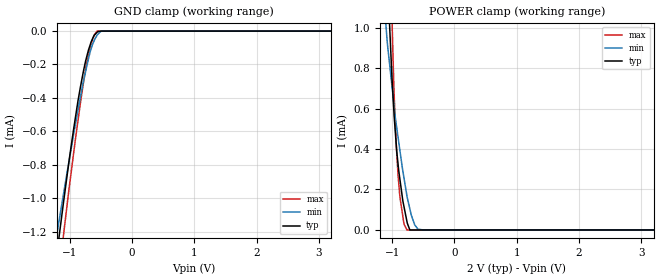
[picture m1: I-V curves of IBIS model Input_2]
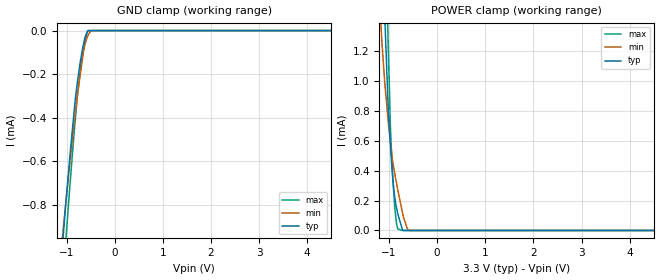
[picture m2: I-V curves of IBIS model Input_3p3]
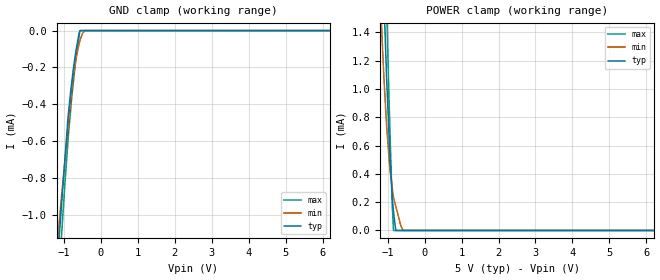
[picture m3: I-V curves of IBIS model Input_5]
|Texas Instruments Incorporated
|12-Bit, Octal, Ultralow Glitch, Voltage Output Digital to Analog Converter
| Marketing part#   Digital Voltage Range   Package-type   #pins
| DAC7558IRHBR   2.7 to 5.5V   QFN   32
| DAC7558IRHBRG4   2.7 to 5.5V   QFN   32
| DAC7558IRHBT   2.7 to 5.5V   QFN   32
| DAC7558IRHBTG4   2.7 to 5.5V   QFN   32
[IBIS Ver]   3.2
[File name]   dac7558.ibs
|SIMDE Ver   V2.0 - 201002 - RHL4 - Build 372
[File Rev]   1.1
[Date]   August 03, 2010
[Source]
|   Texas Instruments Incorporated.
|   Analog-eLab Design Center, HPA
|   12500 TI Blvd
|   Dallas, TX -75243
|   e-mail: elab_ibis@list.ti.com
|   -Model generated from simulations in TISPICE
[Notes]   Revision History:
|   Rev 1.0: 07/13/2010
|   - Initial version of the model
|   - Model generated from simulations in TISPICE
|   - Model matched to SPICE simulation
|   - Models with names containing a trailing 3p3 contain
|   the models for 3.3V [3.0V and 3.6V]. Models with names
|   with trailing 5 contain the models for 5.0V [4.5V and
|   5.5V] operation. And Models with names containing trailing
|   2 contain models for 2V [1.8V and 2.2V].
|   - C_comp although listed in numerical order of value are
|   obtained from varying PVT conditions. For PVT conditions for
|   each specific value refer the buffer description under
|   respective [Model]. IBIS model user is responsible for using
|   appropriate C_comp to simulate for Signal Integrity.
|   Rev 1.1: 08/03/2010
|   - Corrected details under [Package] section.
|   - Added [Model Spec] in all input models
|   - Added comments for C_comp and [Temperature Range].
|   - Added C_comp for ON and HIGH IMPEDANCE states for
|   all 3-state buffers.
|   - Corrected Vinl and Vinh values in Input_3p3 and Input_5
|   models as per datasheet.
|   - Removed extra data points beyond -VDDtyp & 2*VDDtyp in
|   IV data.
|   - Corrected I-V/V-t mismatches for output models.
|   - Voltage range and Power clamp range for TERM changed to
|   1.8v to 5.5v
[Disclaimer]
| This model is designed as an aid for customers of Texas Instruments.
| TI and its licensors and suppliers make no warranties, either expressed
| or implied, with respect to this  model, including the warranties of
| merchantability or fitness for a particular purpose. The model is
| provided solely on an "as is" basis. The entire risk as to its quality
| and performance is with the customer.
[Copyright]
|(C) Copyright 2010 Texas Instruments Incorporated.All rights reserved.
|   DAC7558
[Component]   DAC7558
[Manufacturer]  TI
[Package]   | 32 QFN - RHB Package
|   typ   min   max
R_pkg   0.06441   0.03921   0.07733
L_pkg   1.08058nH   0.96917nH   1.25858nH
C_pkg   0.11700pF   0.10514pF   0.14494pF
|-------------------------PINS------------------------------------------------
[Pin]  signal_name model_name   R_pin   L_pin   C_pin
1   VFBA   TERM   0.07176   1.15274nH   0.10934pF
2   VOUTA   NC   0.06437   1.01850nH   0.10917pF
3   VOUTB   NC   0.06397   1.01087nH   0.10804pF
4   VFBB   TERM   0.06152   0.96917nH   0.10514pF
5   VFBC   TERM   0.06152   0.96920nH   0.10518pF
6   VOUTC   NC   0.06450   1.02377nH   0.10878pF
7   VOUTD   NC   0.06495   1.03230nH   0.11002pF
8   VFBD   TERM   0.07270   1.17584nH   0.11059pF
9   VREF2   NC   0.03936   0.98832nH   0.14273pF
10   SDO   OUTPUT   0.07733   1.25858nH   0.12438pF
11   IOVDD   POWER   0.03721   0.90944nH   0.14943pF
12   DGND   GND   0.03782   0.92935nH   0.14861pF
13   SDIN   INPUT   0.07429   1.20279nH   0.11973pF
14   SCLK   INPUT   0.07311   1.18150nH   0.11929pF
15   _SYNC   INPUT   0.07480   1.21269nH   0.12223pF
16   VREF3   NC   0.03924   0.98339nH   0.14461pF
17   VFBE   TERM   0.07270   1.17584nH   0.11064pF
18   VOUTE   NC   0.06495   1.03229nH   0.11003pF
19   VOUTF   NC   0.06450   1.02377nH   0.10879pF
20   VFBF   TERM   0.06152   0.96920nH   0.10518pF
21   VFBG   TERM   0.06152   0.96917nH   0.10514pF
22   VOUTG   NC   0.06397   1.01088nH   0.10803pF
23   VOUTH   NC   0.06437   1.01851nH   0.10917pF
24   VFBH   TERM   0.07176   1.15274nH   0.10941pF
25   VREF4   NC   0.03921   0.97897nH   0.14445pF
26   DCEN   INPUT   0.07480   1.20388nH   0.12194pF
27   _PD   INPUT   0.07311   1.17249nH   0.11840pF
28   VDD   POWER   0.03582   0.84776nH   0.15059pF
29   AGND   GND   0.02469   0.77509nH   0.17946pF
30   RSTSEL   INPUT   0.07315   1.17310nH   0.11837pF
31   _RST   INPUT   0.07509   1.20907nH   0.12231pF
32   VREF1   NC   0.03945   0.98680nH   0.14494pF
|   Model Selectors
[Model Selector]   INPUT
Input_2   2.0V digital input
Input_3p3   3.3V digital input
Input_5   5.0V digital input
[Model Selector]   OUTPUT
Output_2   2.0V digital tristate output
Output_3p3   3.3V digital tristate output
Output_5   5.0V digital tristate output
|   TERM Model
[Model] TERM
Model_type Terminator
C_comp   1.0e-20F   1.0e-20F   1.0e-20F
| variable   typ   min   max
[Voltage Range]   3.3V   1.8V   5.5V
[POWER Clamp Reference]  3.3V   1.8V   5.5V
[GND Clamp Reference]   0.0V   0.0V   0.0V
|Operating Temperature
|Ambient Temperature   25   105   -40
|Junction Temperature
[Temperature Range]   25   105   -40
| Models and submodels in the file (7): Input_2 (Input), Input_3p3 (Input), Input_5 (Input), Output_2 (3-state), Output_3p3 (3-state), Output_5 (3-state), TERM (Terminator)
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|   INPUT 2.0V Model
[Model]   Input_2
Model_type   Input
Vinl = 0
Vinh = 2.0
|   typ   min   max
|   (nom PVT)   (fast PVT)  (slow PVT)
|Average
C_comp   5.289e-13   5.087e-13   5.331e-13
|Where nom PVT is Nominal Process, 2V, 25C
|   fast PVT is Strong Process, 2.2V, -40C
|   slow PVT is Weak Process, 1.8V, 105C
[Model Spec]
Vinl   0   0   0
Vinh   2.0   1.8   2.2
[Voltage Range]   2   1.8   2.2
|Ambient Temperature   25   105   -40
|Junction Temperature
[Temperature Range]   25   105   -40
[Power Clamp Reference]   2   1.8   2.2
[GND Clamp Reference]   0   0   0
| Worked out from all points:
|   GND clamp passes 1 mA (typ) near -1.09 V on its own axis
|   POWER clamp passes 1 mA (typ) near -1.04 V on its own axis
[GND Clamp]
|   Voltage   I(typ)   I(min)   I(max)
-2V       -3.773mA   -3.073mA   -4.859mA
-1.198V   -1.313mA   -1.199mA   -1.559mA
-1.166V   -1.22mA    -1.127mA   -1.446mA
-1.096V   -1.017mA   -969.5uA   -1.211mA
-996mV    -740.9uA   -748.6uA   -904.1uA
-868mV    -421.9uA   -476.5uA   -540.8uA
-759.2mV  -205.8uA   -268.6uA   -262.6uA
-719.6mV  -144.4uA   -201.6uA   -175.3uA
-660.2mV  -71.04uA   -111.3uA   -82.3uA
-558.2mV  -6.611uA   -23.75uA   0A
-462.8mV  0A         0A         0A
4V        0A         0A         0A
[POWER Clamp]
|   Voltage   I(typ)   I(min)   I(max)
-2V       12.81mA    9.404mA    16.72mA
-1.098V   1.46mA     1.003mA    2.207mA
-1.052V   1.086mA    850.6uA    1.616mA
-1.025V   904.8uA    774.5uA    1.291mA
-1.002V   747.7uA    707.6uA    1.032mA
-957.2mV  517.2uA    579.4uA    580.3uA
-904.4mV  322.3uA    456.1uA    266.6uA
-809.8mV  114.9uA    256.2uA    29.07uA
-761.6mV  40.2uA     166.2uA    0A
-637.4mV  0A         24.9uA     0A
-491.6mV  0A         0A         0A
4V        0A         0A         0A
|   INPUT 3.3V Model
[Model]   Input_3p3
Model_type   Input
Vinl = 0.99
Vinh = 2.31
|   typ   min   max
|   (nom PVT)   (fast PVT)  (slow PVT)
|Average
C_comp   5.026e-13   4.615e-13   5.117e-13
|Where nom PVT is Nominal Process, 3.3V, 25C
|   fast PVT is Strong Process, 3.6V, -40C
|   slow PVT is Weak Process, 3.0V, 105C
[Model Spec]
Vinl   0.99   0.9   1.08
Vinh   2.31   2.1   2.52
[Voltage Range]   3.3   3   3.6
|Ambient Temperature   25   105   -40
|Junction Temperature
[Temperature Range]   25   105   -40
[Power Clamp Reference]   3.3   3   3.6
[GND Clamp Reference]   0   0   0
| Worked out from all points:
|   GND clamp passes 1 mA (typ) near -1.09 V on its own axis
|   POWER clamp passes 1 mA (typ) near -1.04 V on its own axis
[GND Clamp]
|   Voltage   I(typ)   I(min)   I(max)
-3.3V     -7.87mA    -6.18mA    -10.49mA
-1.136V   -1.137mA   -1.06mA    -1.344mA
-1.043V   -869.1uA   -851.3uA   -1.043mA
-1.016V   -796uA     -793uA     -965.3uA
-927.6mV  -570.2uA   -602.2uA   -704.9uA
-825mV    -329.3uA   -390.9uA   -425.6uA
-772.2mV  -232.4uA   -297.8uA   -290.7uA
-697.2mV  -121.4uA   -173.8uA   -154.5uA
-645mV    -59.97uA   -92.43uA   -82.6uA
-554.4mV  0A         -22.62uA   0A
-466.8mV  0A         0A         0A
6.6V      0A         0A         0A
[POWER Clamp]
|   Voltage   I(typ)   I(min)   I(max)
-3.3V     30.52mA    23.75mA    38.67mA
-1.165V   2.169mA    1.36mA     3.176mA
-1.086V   1.411mA    976.9uA    2.1mA
-1.057V   1.164mA    874.8uA    1.729mA
-1.02V    842uA      742uA      1.278mA
-970.8mV  563uA      589.3uA    689.2uA
-924mV    352.6uA    461.9uA    363uA
-877.2mV  213.9uA    374.9uA    141.1uA
-819.6mV  113.6uA    273.2uA    11.09uA
-722.4mV  5.068uA    122.4uA    0A
-574.8mV  0A         0A         0A
6.6V      0A         0A         0A
|   INPUT 5.0V Model
[Model]   Input_5
Model_type   Input
Vinl = 1.5
Vinh = 3.5
|   typ   min   max
|   (nom PVT)   (fast PVT)  (slow PVT)
|Average
C_comp   4.311e-13   4.270e-13   4.887e-13
|Where nom PVT is Nominal Process, 5V, 25C
|   fast PVT is Strong Process, 5.5V, -40C
|   slow PVT is Weak Process, 4.5V, 105C
[Model Spec]
Vinl   1.5   1.35   1.65
Vinh   3.5   3.15   3.85
[Voltage Range]   5   4.5   5.5
|Ambient Temperature   25   105   -40
|Junction Temperature
[Temperature Range]   25   105   -40
[Power Clamp Reference]   5   4.5   5.5
[GND Clamp Reference]   0   0   0
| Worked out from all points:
|   GND clamp passes 1 mA (typ) near -1.08 V on its own axis
|   POWER clamp passes 1 mA (typ) near -1.02 V on its own axis
[GND Clamp]
|   Voltage   I(typ)   I(min)   I(max)
-5V       -13.27mA   -10.27mA   -17.9mA
-1.172V   -1.238mA   -1.141mA   -1.465mA
-1.079V   -983.7uA   -930uA     -1.154mA
-1.062V   -940.1uA   -894uA     -1.105mA
-895mV    -484.4uA   -542.9uA   -613uA
-815mV    -326.2uA   -375.2uA   -422uA
-761mV    -235.4uA   -268.3uA   -309.3uA
-666.5mV  -99.98uA   -146.1uA   -140.8uA
-595mV    -21.44uA   -77.84uA   -38.12uA
-558.5mV  0A         -49.68uA   0A
-430mV    0A         0A         0A
10V       0A         0A         0A
[POWER Clamp]
|   Voltage   I(typ)   I(min)   I(max)
-5V       53.94mA    42.83mA    67.6mA
-1.177V   2.294mA    1.521mA    3.356mA
-1.15V    2.04mA     1.354mA    3.001mA
-1.099V   1.609mA    1.065mA    2.382mA
-1.062V   1.332mA    893.4uA    1.95mA
-1.025V   1.056mA    727.4uA    1.563mA
-979.5mV  776.4uA    571.1uA    1.087mA
-880.5mV  265.9uA    306.1uA    205.4uA
-837.5mV  124.6uA    228.2uA    0A
-780mV    0A         170.3uA    0A
-572.5mV  0A         0A         0A
10V       0A         0A         0A
